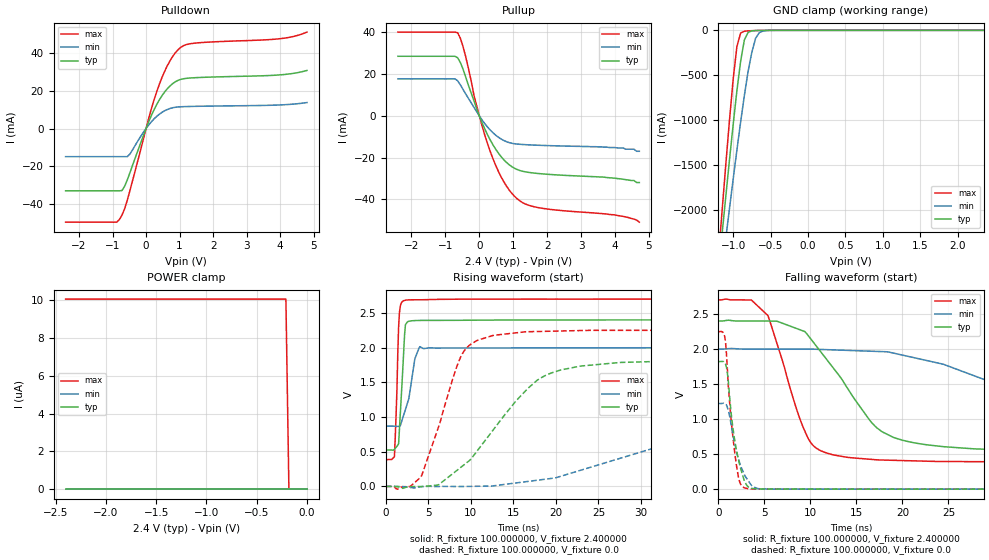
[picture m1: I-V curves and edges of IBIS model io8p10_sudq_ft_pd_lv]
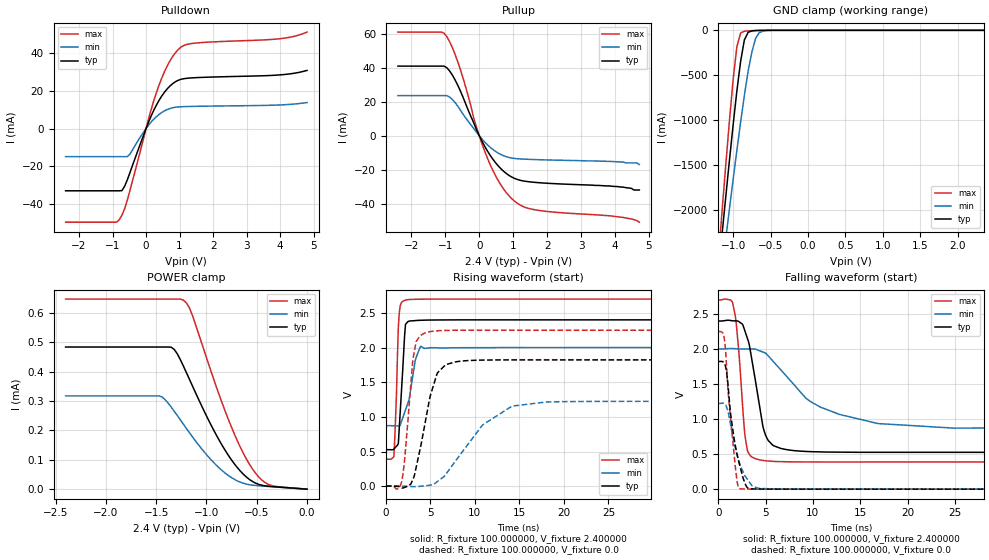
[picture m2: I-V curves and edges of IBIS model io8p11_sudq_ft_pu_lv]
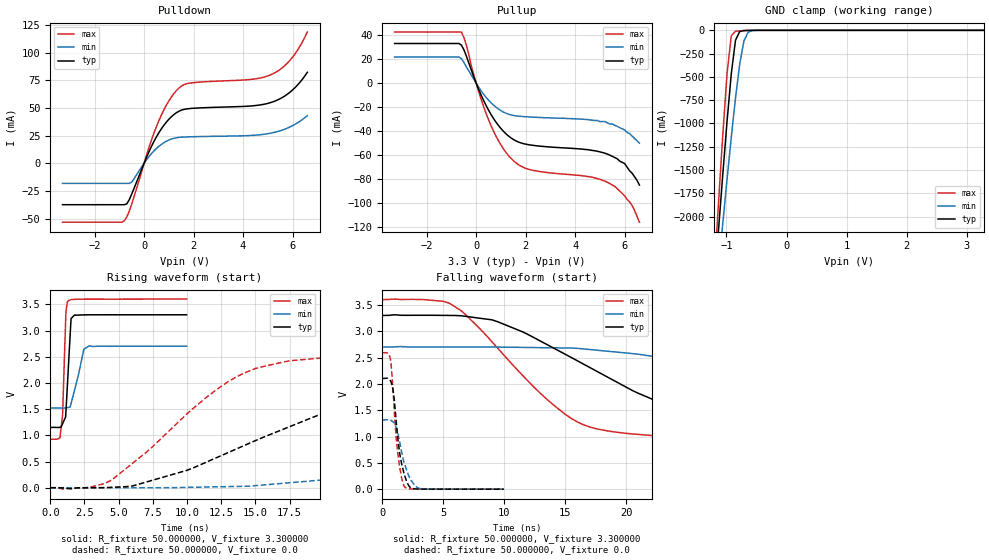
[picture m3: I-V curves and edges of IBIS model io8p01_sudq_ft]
| IBIS file stm32f303x6x8_334_lqfp48.ibs
[IBIS ver] 4.2
[File name] stm32f303x6x8_334_lqfp48.ibs
[File Rev] 1
[Date]  29-09-2025
[Source] Data Created at STMicroelectronics
[Notes]  File originated from ELDO simulations.
[Disclaimer]  This information is for modeling purpose only and is
   not guaranted. The information is subject to change without
   notice.
[Copyright] Copyright 2025 STMicroelectronics Inc.
|   Component stm32f303x6x8_334_lqfp48
[Component] stm32f303x6x8_334_lqfp48
[Manufacturer] STMicroelectronics
[Package]
| variable   typ   min   max
R_pkg   0.0   0.0   0.0
L_pkg   0.0H   0.0H   0.0H
C_pkg   0.0F   0.0F   0.0F
[Pin]  signal_name   model_name   R_pin   L_pin   C_pin
1 VBAT POWER 0.053 3.42534E-09 9.041E-14
2 PC13 io8p_sudq_tc 0.048377332 2.91404E-09 6.443E-14
3 PC14 io8p_sudq_tc 0.044678997 2.50442E-09 4.365E-14
4 PC15 io8p_sudq_tc 0.041905328 2.19704E-09 2.807E-14
5 PF0 io8p_sudq_ft 0.040056325 1.9919E-09 1.769E-14
6 PF1 io8p_sudq_ft 0.03913 1.89021E-09 1.24625E-14
7 NRST ioreset_tc_v33 0.03913 1.89021E-09 1.24625E-14
8 VSSA GND 0.040057312 1.98992E-09 1.775E-14
9 VDDA POWER 0.041906973 2.19374E-09 2.817E-14
10 PA0 io8p_sudq_tc 0.0446813 2.4998E-09 4.379E-14
11 PA1 io8p_sudq_tc 0.048380293 2.9081E-09 6.461E-14
12 PA2 io8p_sudq_tc 0.053 3.42534E-09 9.041E-14
13 PA3 io8p_sudq_tc 0.053 3.42534E-09 9.041E-14
14 PA4 io8p_sudq_tc 0.048377332 2.91404E-09 6.443E-14
15 PA5 io8p_sudq_tc 0.044678997 2.50442E-09 4.365E-14
16 PA6 io8p_sudq_tc 0.041905328 2.19704E-09 2.807E-14
17 PA7 io8p_sudq_tc 0.040056325 1.9919E-09 1.769E-14
18 PB0 io8p_sudq_tc 0.03913 1.89021E-09 1.24625E-14
19 PB1 io8p_sudq_tc 0.03913 1.89021E-09 1.24625E-14
20 PB2 io8p_sudq_tc 0.040057312 1.98992E-09 1.775E-14
21 PB10 io8p_sudq_tc 0.041906973 2.19374E-09 2.817E-14
22 PB11 io8p_sudq_tc 0.0446813 2.4998E-09 4.379E-14
23 VSS GND 0.048380293 2.9081E-09 6.461E-14
24 VDD POWER 0.053 3.42534E-09 9.041E-14
25 PB12 io8p_sudq_tc 0.053 3.42534E-09 9.041E-14
26 PB13 io8p_sudq_tc 0.048377332 2.91404E-09 6.443E-14
27 PB14 io8p_sudq_tc 0.044678997 2.50442E-09 4.365E-14
28 PB15 io8p_sudq_tc 0.041905328 2.19704E-09 2.807E-14
29 PA8 io8p_sudq_ft 0.040056325 1.9919E-09 1.769E-14
30 PA9 io8p_sudq_ft 0.03913 1.89021E-09 1.24625E-14
31 PA10 io8p_sudq_ft 0.03913 1.89021E-09 1.24625E-14
32 PA11 io8p_sudq_ft 0.040057312 1.98992E-09 1.775E-14
33 PA12 io8p_sudq_ft 0.041906973 2.19374E-09 2.817E-14
34 PA13 io8p_sudq_ft 0.0446813 2.4998E-09 4.379E-14
35 VSS GND 0.048380293 2.9081E-09 6.461E-14
36 VDD POWER 0.053 3.42534E-09 9.041E-14
37 PA14 io8p_wsudqh_i2c_ft 0.053 3.42534E-09 9.041E-14
38 PA15 io8p_wsudqh_i2c_ft 0.048377332 2.91404E-09 6.443E-14
39 PB3 io8p_sudq_ft 0.044678997 2.50442E-09 4.365E-14
40 PB4 io8p_sudq_ft 0.041905328 2.19704E-09 2.807E-14
41 PB5 io8p_sudq_ft 0.040056325 1.9919E-09 1.769E-14
42 PB6 io8p_wsudqh_i2c_ft 0.03913 1.89021E-09 1.24625E-14
43 PB7 io8p_wsudqh_i2c_ft 0.03913 1.89021E-09 1.24625E-14
44 BOOT0 vpp_test_hv 0.040057312 1.98992E-09 1.775E-14
45 PB8 io8p_wsudqh_i2c_ft 0.041906973 2.19374E-09 2.817E-14
46 PB9 io8p_wsudqh_i2c_ft 0.0446813 2.4998E-09 4.379E-14
47 VSS_PLUS_1 GND 0.048380293 2.9081E-09 6.461E-14
48 VDD POWER 0.053 3.42534E-09 9.041E-14
[Model Selector] io8p_sudq_ft
io8p01_sudq_ft_pd_lv  "SPEED01 2P0V, PD=40kOhm"
io8p01_sudq_ft_pu_lv  "SPEED01 2P0V, PU=40kOhm"
io8p01_sudq_ft_lv  "SPEED01 2P0V"
io8p10_sudq_ft_pd_lv  "SPEED10 2P0V, PD=40kOhm"
io8p10_sudq_ft_pu_lv  "SPEED10 2P0V, PU=40kOhm"
io8p10_sudq_ft_lv  "SPEED10 2P0V"
io8p11_sudq_ft_pd_lv  "SPEED11 2P0V, PD=40kOhm"
io8p11_sudq_ft_pu_lv  "SPEED11 2P0V, PU=40kOhm"
io8p11_sudq_ft_lv  "SPEED11 2P0V"
io8p01_sudq_ft_pd  "SPEED01, PD=40kOhm"
io8p01_sudq_ft_pu  "SPEED01, PU=40kOhm"
io8p01_sudq_ft  "SPEED01"
io8p10_sudq_ft_pd  "SPEED10, PD=40kOhm"
io8p10_sudq_ft_pu  "SPEED10, PU=40kOhm"
io8p10_sudq_ft  "SPEED10"
io8p11_sudq_ft_pd  "SPEED11, PD=40kOhm"
io8p11_sudq_ft_pu  "SPEED11, PU=40kOhm"
io8p11_sudq_ft  "SPEED11"
[Model Selector] io8p_sudq_tc
io8p01_sudq_tc_pd_lv  "SPEED01 2P0V, PD=40kOhm"
io8p01_sudq_tc_pu_lv  "SPEED01 2P0V, PU=40kOhm"
io8p01_sudq_tc_lv  "SPEED01 2P0V"
io8p10_sudq_tc_pd_lv  "SPEED10 2P0V, PD=40kOhm"
io8p10_sudq_tc_pu_lv  "SPEED10 2P0V, PU=40kOhm"
io8p10_sudq_tc_lv  "SPEED10 2P0V"
io8p11_sudq_tc_pd_lv  "SPEED11 2P0V, PD=40kOhm"
io8p11_sudq_tc_pu_lv  "SPEED11 2P0V, PU=40kOhm"
io8p11_sudq_tc_lv  "SPEED11 2P0V"
io8p01_sudq_tc_pd  "SPEED01, PD=40kOhm"
io8p01_sudq_tc_pu  "SPEED01, PU=40kOhm"
io8p01_sudq_tc  "SPEED01"
io8p10_sudq_tc_pd  "SPEED10, PD=40kOhm"
io8p10_sudq_tc_pu  "SPEED10, PU=40kOhm"
io8p10_sudq_tc  "SPEED10"
io8p11_sudq_tc_pd  "SPEED11, PD=40kOhm"
io8p11_sudq_tc_pu  "SPEED11, PU=40kOhm"
io8p11_sudq_tc  "SPEED11"
[Model Selector] io8p_wsudqh_i2c_ft
io8p_wsudqh_i2c_ft_lv_pd  "General purpose IO with I2C capability on. 5V tolerant. 1.8V range with pull down"
io8p_wsudqh_i2c_ft_lv_pu  "General purpose IO with I2C capability on. 5V tolerant. 1.8V range with pull up"
io8p_wsudqh_i2c_ft_lv  "General purpose IO with I2C capability on. 5V tolerant. 1.8V range"
io8p_wsudqh_i2c_ft_pd  "General purpose IO with I2C capability on. 5V tolerant. 3.3V range with pull down"
io8p_wsudqh_i2c_ft_pu  "General purpose IO with I2C capability on. 5V tolerant. 3.3V range with pull up"
io8p_wsudqh_i2c_ft_i2c  "General purpose IO with I2C capability on. 5V tolerant. 3.3V range"
[Model Selector] ioreset_tc_v33
ioreset_tc_v33_pu_lv  "IORESET 2V + PU=40kOhm"
ioreset_tc_v33_nopu_lv  "IORESET 2V"
ioreset_tc_v33_pu  "IORESET + PU=40kOhm"
ioreset_tc_v33_nopu  "IORESET"
[Model Selector] vpp_test_hv
vpp_test_hv_3p3  "Input Buffer"
vpp_test_hv_2p4  "Input Buffer 2P0V"
| Models and submodels in the file (48): io8p01_sudq_ft_pd_lv (I/O), io8p01_sudq_ft_pu_lv (I/O), io8p01_sudq_ft_lv (I/O), io8p10_sudq_ft_pd_lv (I/O), io8p10_sudq_ft_pu_lv (I/O), io8p10_sudq_ft_lv (I/O), io8p11_sudq_ft_pd_lv (I/O), io8p11_sudq_ft_pu_lv (I/O), io8p11_sudq_ft_lv (I/O), io8p01_sudq_ft_pd (I/O), io8p01_sudq_ft_pu (I/O), io8p01_sudq_ft (I/O), io8p10_sudq_ft_pd (I/O), io8p10_sudq_ft_pu (I/O), io8p10_sudq_ft (I/O), io8p11_sudq_ft_pd (I/O), io8p11_sudq_ft_pu (I/O), io8p11_sudq_ft (I/O), io8p01_sudq_tc_pd_lv (I/O), io8p01_sudq_tc_pu_lv (I/O), io8p01_sudq_tc_lv (I/O), io8p10_sudq_tc_pd_lv (I/O), io8p10_sudq_tc_pu_lv (I/O), io8p10_sudq_tc_lv (I/O), io8p11_sudq_tc_pd_lv (I/O), io8p11_sudq_tc_pu_lv (I/O), io8p11_sudq_tc_lv (I/O), io8p01_sudq_tc_pd (I/O), io8p01_sudq_tc_pu (I/O), io8p01_sudq_tc (I/O), io8p10_sudq_tc_pd (I/O), io8p10_sudq_tc_pu (I/O), io8p10_sudq_tc (I/O), io8p11_sudq_tc_pd (I/O), io8p11_sudq_tc_pu (I/O), io8p11_sudq_tc (I/O), io8p_wsudqh_i2c_ft_lv_pd (I/O), io8p_wsudqh_i2c_ft_lv_pu (I/O), io8p_wsudqh_i2c_ft_lv (I/O), io8p_wsudqh_i2c_ft_pd (I/O), io8p_wsudqh_i2c_ft_pu (I/O), io8p_wsudqh_i2c_ft_i2c (I/O), ioreset_tc_v33_pu_lv (I/O_open_drain), ioreset_tc_v33_nopu_lv (I/O_open_drain), ioreset_tc_v33_pu (I/O_open_drain), ioreset_tc_v33_nopu (I/O_open_drain), vpp_test_hv_2p4 (Input), vpp_test_hv_3p3 (Input)
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|   Model io8p10_sudq_ft_pd_lv
[Model]  io8p10_sudq_ft_pd_lv
Model_type I/O
Polarity   Non-Inverting
Enable   Active-Low
Vinl =   0.720000V
Vinh =   1.680000V
Vmeas =  1.200000V
Cref =   50.000000pF
Rref =   100.000000M
Vref =   0.0V
C_comp   1.970100pF   1.887900pF   2.069400pF
[Temperature Range]   25.000000   0.125000k   -40.000000
[Pullup Reference]   2.400000V   2.000000V   2.700000V
[Pulldown Reference]   0.0V   0.0V   0.0V
[POWER Clamp Reference]   2.400000V   2.000000V   2.700000V
[GND Clamp Reference]   0.0V   0.0V   0.0V
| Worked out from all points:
|   slope of the pulldown table from 0 to 0.36 V, typ, clamps not added: 25.5 ohm
|   slope of the pullup table from 0 to 0.36 V, typ, clamps not added: 28.4 ohm
|   GND clamp passes 1 mA (typ) near -0.64 V on its own axis
|   rising waveform, R_fixture 100.000000, V_fixture 2.400000: 20-80 % time 501ps typ, 1.06ns min, 337ps max; typ from 0.525 V to 2.4 V
|   rising waveform, R_fixture 100.000000, V_fixture 0.0: 20-80 % time 7.37ns typ, 21.8ns min, 3.53ns max; typ from 0 V to 1.82 V
|   falling waveform, R_fixture 100.000000, V_fixture 2.400000: 20-80 % time 6.27ns typ, 17.5ns min, 3.34ns max; typ from 2.4 V to 0.525 V
|   falling waveform, R_fixture 100.000000, V_fixture 0.0: 20-80 % time 1.15ns typ, 1.39ns min, 910ps max; typ from 1.82 V to 0 V
[Pulldown]
|Voltage   I(typ)   I(min)   I(max)
-2.4V     -33.16mA   -14.98mA   -49.86mA
-880mV    -33.16mA   -14.98mA   -49.86mA
-800mV    -33.16mA   -14.98mA   -48.55mA
-640mV    -30.75mA   -14.98mA   -42.76mA
-480mV    -23.43mA   -13.57mA   -32.92mA
80mV      3.651mA    1.905mA    5.506mA
400mV     15.37mA    7.665mA    23.73mA
720mV     22.75mA    10.69mA    36.23mA
1.04V     26.18mA    11.57mA    43.27mA
1.52V     27.09mA    11.81mA    45.55mA
4V        28.55mA    12.55mA    47.81mA
4.8V      30.9mA     13.81mA    51.31mA
[Pullup]
|Voltage   I(typ)   I(min)   I(max)
-2.4V     28.56mA    17.75mA    40.16mA
-720mV    28.56mA    17.75mA    40.16mA
-640mV    27.85mA    16.83mA    39.87mA
-480mV    22.39mA    12.66mA    33.22mA
-80mV     3.427mA    2.067mA    4.957mA
160mV     -6.219mA   -3.715mA   -9.137mA
320mV     -11.51mA   -6.781mA   -16.98mA
720mV     -21mA      -11.8mA    -31.53mA
1.12V     -25.77mA   -13.54mA   -39.82mA
1.76V     -27.69mA   -14.12mA   -44.07mA
4V        -29.9mA    -15.2mA    -47.5mA
4.72V     -32mA      -17mA      -51mA
[GND_clamp]
|Voltage   I(typ)   I(min)   I(max)
-2.4V     -9.788A    -9.782A    -9.734A
-1.2V     -2.718A    -3.021A    -2.568A
-1.15V    -2.29A     -2.675A    -2.036A
-1.1V     -1.868A    -2.333A    -1.515A
-1.05V    -1.454A    -1.995A    -1.012A
-950mV    -674.5mA   -1.337A    -180.6mA
-900mV    -345.2mA   -1.023A    -29.74mA
-850mV    -106.4mA   -726mA     -10.14mA
-750mV    -6.411mA   -244mA     -4.042mA
-700mV    -2.572mA   -88.62mA   -2.346mA
-600mV    -429.6uA   -7.75mA    -383.5uA
2.35V     59.77uA    46.33uA    66.89uA
[POWER_clamp]
|Voltage   I(typ)   I(min)   I(max)
-2.4V     0A         0A         10.06uA
-210mV    0A         0A         10.06uA
-180mV    0A         0A         0A
0V        0A         0A         0A
[Ramp]
| variable   typ   min   max
dV/dt_r  1.09206/7.36205n   0.73212/21.76780n   1.34880/3.52140n
dV/dt_f  1.12434/6.26286n   0.67629/17.46251n   1.38699/3.33301n
R_load = 100.000000
[Rising Waveform]
R_fixture= 100.000000
V_fixture= 2.400000
V_fixture_min= 2.000000
V_fixture_max= 2.700000
|time   V(typ)   V(min)   V(max)
0s        524.8mV    868.7mV    387.2mV
1.001ns   532.8mV    867mV      426.6mV
1.301ns   578.6mV    865.5mV    1.387V
1.502ns   616.5mV    864.9mV    2.303V
1.702ns   1.053V     875.4mV    2.602V
2.102ns   1.953V     1.031V     2.676V
2.302ns   2.331V     1.108V     2.683V
3.403ns   2.389V     1.835V     2.689V
4.004ns   2.392V     2.014V     2.689V
49.85ns   2.399V     1.999V     2.699V
[Rising Waveform]
R_fixture= 100.000000
V_fixture= 0.0
V_fixture_min= 0.0
V_fixture_max= 0.0
|time   V(typ)   V(min)   V(max)
0s        1.768nV    15.89nV    1.355nV
2.803ns   -3.26mV    -14.06mV   -1.551mV
4.204ns   -1.822mV   -2.484mV   153.2mV
6.206ns   24.43mV    -1.172mV   860.8mV
8.809ns   274.4mV    -1.373mV   1.867V
12.61ns   812.3mV    7.914mV    2.175V
17.82ns   1.532V     89.58mV    2.232V
23.02ns   1.735V     237.2mV    2.246V
50.05ns   1.82V      1.08V      2.248V
99.7ns    1.82V      1.221V     2.248V
[Falling Waveform]
R_fixture= 100.000000
V_fixture= 2.400000
V_fixture_min= 2.000000
V_fixture_max= 2.700000
|time   V(typ)   V(min)   V(max)
0s        2.399V     1.999V     2.699V
3.604ns   2.399V     1.998V     2.698V
5.405ns   2.398V     1.998V     2.475V
9.61ns    2.218V     1.997V     767.5mV
12.61ns   1.708V     1.986V     485.9mV
17.62ns   835.2mV    1.963V     416.1mV
24.42ns   606.3mV    1.782V     394.4mV
31.83ns   557.1mV    1.421V     389.7mV
47.25ns   529mV      987.2mV    387.3mV
99.7ns    524.8mV    868.7mV    387.2mV
[Falling Waveform]
R_fixture= 100.000000
V_fixture= 0.0
V_fixture_min= 0.0
V_fixture_max= 0.0
|time   V(typ)   V(min)   V(max)
0s        1.82V      1.221V     2.248V
700.7ps   1.8V       1.221V     2.179V
800.8ps   1.783V     1.214V     2.096V
1.001ns   1.653V     1.163V     1.703V
1.401ns   1.09V      921.9mV    991.5mV
1.802ns   688.2mV    647.3mV    514.6mV
2.302ns   364.8mV    386.2mV    116.7mV
2.903ns   104.8mV    188.7mV    16.24mV
4.705ns   2.13mV     3.846mV    2.055mV
49.85ns   1.768nV    15.89nV    1.355nV
|   Model io8p11_sudq_ft_pu_lv
[Model]  io8p11_sudq_ft_pu_lv
Model_type I/O
Polarity   Non-Inverting
Enable   Active-Low
Vinl =   0.720000V
Vinh =   1.680000V
Vmeas =  1.200000V
Cref =   50.000000pF
Rref =   100.000000M
Vref =   0.0V
C_comp   1.970100pF   1.887900pF   2.069400pF
[Temperature Range]   25.000000   0.125000k   -40.000000
[Pullup Reference]   2.400000V   2.000000V   2.700000V
[Pulldown Reference]   0.0V   0.0V   0.0V
[POWER Clamp Reference]   2.400000V   2.000000V   2.700000V
[GND Clamp Reference]   0.0V   0.0V   0.0V
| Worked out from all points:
|   slope of the pulldown table from 0 to 0.36 V, typ, clamps not added: 25.5 ohm
|   slope of the pullup table from 0 to 0.36 V, typ, clamps not added: 28.4 ohm
|   GND clamp passes 1 mA (typ) near -0.64 V on its own axis
|   rising waveform, R_fixture 100.000000, V_fixture 2.400000: 20-80 % time 508ps typ, 1.05ns min, 337ps max; typ from 0.527 V to 2.4 V
|   rising waveform, R_fixture 100.000000, V_fixture 0.0: 20-80 % time 1.8ns typ, 4.87ns min, 863ps max; typ from 0.001 V to 1.82 V
|   falling waveform, R_fixture 100.000000, V_fixture 2.400000: 20-80 % time 1.39ns typ, 6.08ns min, 775ps max; typ from 2.4 V to 0.527 V
|   falling waveform, R_fixture 100.000000, V_fixture 0.0: 20-80 % time 1.17ns typ, 1.4ns min, 853ps max; typ from 1.82 V to 0.001 V
[Pulldown]
|Voltage   I(typ)   I(min)   I(max)
-2.4V     -33.16mA   -14.98mA   -49.86mA
-880mV    -33.16mA   -14.98mA   -49.86mA
-800mV    -33.16mA   -14.98mA   -48.55mA
-640mV    -30.75mA   -14.98mA   -42.77mA
-480mV    -23.43mA   -13.57mA   -32.92mA
80mV      3.651mA    1.905mA    5.506mA
400mV     15.37mA    7.665mA    23.73mA
720mV     22.75mA    10.69mA    36.23mA
1.04V     26.18mA    11.57mA    43.27mA
1.52V     27.09mA    11.81mA    45.55mA
4V        28.55mA    12.55mA    47.81mA
4.8V      30.9mA     13.81mA    51.31mA
[Pullup]
|Voltage   I(typ)   I(min)   I(max)
-2.4V     41.12mA    23.71mA    61.21mA
-1.12V    41.12mA    23.71mA    61.21mA
-960mV    40.18mA    23.71mA    58.56mA
-800mV    36.01mA    21.55mA    52.29mA
-560mV    26.54mA    15.18mA    39.21mA
-160mV    7.421mA    4.162mA    10.02mA
240mV     -8.977mA   -5.327mA   -13.21mA
640mV     -19.51mA   -11.09mA   -29.16mA
1.04V     -25.15mA   -13.38mA   -38.61mA
1.68V     -27.56mA   -14.07mA   -43.82mA
3.84V     -29.6mA    -15.1mA    -47.2mA
4.72V     -32mA      -17mA      -51mA
[GND_clamp]
|Voltage   I(typ)   I(min)   I(max)
-2.4V     -9.788A    -9.782A    -9.734A
-1.2V     -2.718A    -3.02A     -2.568A
-1.15V    -2.29A     -2.675A    -2.036A
-1.1V     -1.868A    -2.333A    -1.515A
-1.05V    -1.454A    -1.995A    -1.012A
-950mV    -674.5mA   -1.337A    -180.5mA
-900mV    -345.2mA   -1.023A    -29.72mA
-850mV    -106.4mA   -726mA     -10.13mA
-750mV    -6.396mA   -244mA     -4.026mA
-700mV    -2.558mA   -88.61mA   -2.329mA
-600mV    -416uA     -7.739mA   -368uA
2.35V     0A         0A         0A
[POWER_clamp]
|Voltage   I(typ)   I(min)   I(max)
-2.4V     483.8uA    317.4uA    647uA
-1.47V    483.8uA    317.4uA    647uA
-1.32V    475.6uA    265.2uA    647uA
-1.23V    419.7uA    221.6uA    643.3uA
-1.17V    374.8uA    192.7uA    617.6uA
-1.14V    352.1uA    178.7uA    591.9uA
-840mV    147uA      62.15uA    289.6uA
-690mV    72.24uA    27.76uA    162.7uA
-540mV    25.74uA    13.55uA    67.63uA
-450mV    13.38uA    10.75uA    31.36uA
-360mV    9.231uA    8.535uA    12.97uA
0V        0A         0A         0A
[Ramp]
| variable   typ   min   max
dV/dt_r  1.09269/1.79328n   0.73359/4.86832n   1.34926/0.85997n
dV/dt_f  1.12411/1.38607n   0.67669/6.07307n   1.38681/0.77427n
R_load = 100.000000
[Rising Waveform]
R_fixture= 100.000000
V_fixture= 2.400000
V_fixture_min= 2.000000
V_fixture_max= 2.700000
|time   V(typ)   V(min)   V(max)
0s        526.5mV    872.5mV    388.6mV
900.9ps   534.2mV    870.9mV    425.1mV
1.201ns   577.4mV    869.6mV    1.365V
1.401ns   613.7mV    869.2mV    2.295V
1.602ns   1.046V     879.2mV    2.598V
2.202ns   2.333V     1.099V     2.686V
2.603ns   2.381V     1.245V     2.693V
3.303ns   2.389V     1.817V     2.697V
3.904ns   2.394V     2.019V     2.698V
49.85ns   2.4V       2V         2.7V
[Rising Waveform]
R_fixture= 100.000000
V_fixture= 0.0
V_fixture_min= 0.0
V_fixture_max= 0.0
|time   V(typ)   V(min)   V(max)
0s        1.022mV    1.341mV    911uV
1.802ns   -26.21mV   109.9uV    74.5mV
3.103ns   116.7mV    -6.8mV     1.877V
3.403ns   271.6mV    -8.185mV   2.086V
4.505ns   979.1mV    4.99mV     2.215V
5.706ns   1.605V     58.19mV    2.241V
6.707ns   1.752V     167.1mV    2.247V
10.81ns   1.819V     875.7mV    2.25V
14.21ns   1.822V     1.156V     2.25V
49.85ns   1.822V     1.224V     2.25V
[Falling Waveform]
R_fixture= 100.000000
V_fixture= 2.400000
V_fixture_min= 2.000000
V_fixture_max= 2.700000
|time   V(typ)   V(min)   V(max)
0s        2.4V       2V         2.7V
1.502ns   2.403V     2.008V     2.671V
1.902ns   2.401V     2.004V     2.37V
2.903ns   2.224V     2.001V     697.7mV
4.004ns   1.486V     1.995V     432.1mV
5.205ns   712.7mV    1.914V     402.8mV
7.508ns   558.9mV    1.567V     391mV
10.81ns   532.3mV    1.17V      388.6mV
16.82ns   526.7mV    938mV      388.6mV
49.85ns   526.5mV    872.5mV    388.6mV
[Falling Waveform]
R_fixture= 100.000000
V_fixture= 0.0
V_fixture_min= 0.0
V_fixture_max= 0.0
|time   V(typ)   V(min)   V(max)
0s        1.822V     1.224V     2.25V
700.7ps   1.784V     1.216V     2.102V
1.101ns   1.384V     1.072V     1.307V
1.301ns   1.083V     926.1mV    1.012V
1.802ns   627.4mV    595.9mV    327.6mV
2.102ns   434.5mV    435.4mV    35.99mV
2.302ns   325.6mV    349.7mV    5.728mV
3.103ns   17.78mV    137.1mV    2.333mV
4.605ns   2.394mV    9.48mV     1.404mV
49.85ns   1.022mV    1.341mV    911uV
|   Model io8p01_sudq_ft
[Model]  io8p01_sudq_ft
Model_type I/O
Polarity   Non-Inverting
Enable   Active-Low
Vinl =   0.990000V
Vinh =   2.310000V
Vmeas =  1.650000V
Cref =   50.000000pF
Rref =   100.000000M
Vref =   0.0V
C_comp   1.970900pF   1.892300pF   2.063200pF
[Temperature Range]   25.000000   0.125000k   -40.000000
[Pullup Reference]   3.300000V   2.700000V   3.600000V
[Pulldown Reference]   0.0V   0.0V   0.0V
[POWER Clamp Reference]   3.300000V   2.700000V   3.600000V
[GND Clamp Reference]   0.0V   0.0V   0.0V
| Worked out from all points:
|   slope of the pulldown table from 0 to 0.495 V, typ, clamps not added: 20.9 ohm
|   slope of the pullup table from 0 to 0.495 V, typ, clamps not added: 22.2 ohm
|   GND clamp passes 1 mA (typ) near -0.64 V on its own axis
|   rising waveform, R_fixture 50.000000, V_fixture 3.300000: 20-80 % time 269ps typ, 640ps min, 200ps max; typ from 1.15 V to 3.3 V
|   rising waveform, R_fixture 50.000000, V_fixture 0.0: 20-80 % time 12.5ns typ, 30.4ns min, 7.06ns max; typ from 0 V to 2.1 V
|   falling waveform, R_fixture 50.000000, V_fixture 3.300000: 20-80 % time 10.9ns typ, 22.8ns min, 6.88ns max; typ from 3.3 V to 1.15 V
|   falling waveform, R_fixture 50.000000, V_fixture 0.0: 20-80 % time 666ps typ, 862ps min, 543ps max; typ from 2.1 V to 0 V
[Pulldown]
|Voltage   I(typ)   I(min)   I(max)
-3.3V     -37.45mA   -18.2mA    -53.24mA
-800mV    -37.45mA   -18.2mA    -51.9mA
-700mV    -36.7mA    -18.2mA    -48.48mA
-500mV    -27.71mA   -17.01mA   -36.66mA
200mV     10.57mA    6.084mA    14.57mA
500mV     23.91mA    13.38mA    33.24mA
900mV     37.17mA    19.88mA    52.48mA
1.3V      45.55mA    23.01mA    65.5mA
1.8V      49.29mA    23.83mA    72.18mA
5.1V      54.68mA    27.07mA    79.72mA
5.9V      64.2mA     32.82mA    93.01mA
6.6V      82.13mA    42.97mA    118.4mA
[Pullup]
|Voltage   I(typ)   I(min)   I(max)
-3.3V     33.18mA    21.9mA     42.7mA
-600mV    31.87mA    20.57mA    42.7mA
-400mV    22.78mA    13.76mA    31.89mA
100mV     -5.13mA    -3.299mA   -6.952mA
500mV     -22.5mA    -14.16mA   -30.52mA
900mV     -35.28mA   -21.55mA   -48mA
1.4V      -45.55mA   -26.41mA   -62.54mA
2.2V      -51.57mA   -28.22mA   -72.25mA
5.4V      -60mA      -34mA      -83.7mA
6V        -67mA      -39mA      -94mA
6.2V      -73mA      -42mA      -99mA
6.6V      -85mA      -50mA      -116mA
[GND_clamp]
|Voltage   I(typ)   I(min)   I(max)
-3.3V     -9.525A    -9.501A    -9.513A
-1.2V     -2.719A    -3.023A    -2.568A
-1.13V    -2.122A    -2.541A    -1.826A
-1.06V    -1.537A    -2.065A    -1.111A
-990mV    -975.7mA   -1.599A    -462mA
-920mV    -467.4mA   -1.149A    -59mA
-850mV    -106.6mA   -727.3mA   -10.11mA
-780mV    -13.06mA   -365.4mA   -5.254mA
-710mV    -3.045mA   -114.8mA   -2.635mA
-640mV    -943.2uA   -20.16mA   -905.7uA
-570mV    -199.4uA   -3.959mA   -156.8uA
3.28V     0A         0A         0A
[POWER_clamp]
|Voltage   I(typ)   I(min)   I(max)
-3.28V    0A         0A         0A
0V        0A         0A         0A
[Ramp]
| variable   typ   min   max
dV/dt_r  1.26240/12.53718n   0.78948/30.37625n   1.55460/7.05051n
dV/dt_f  1.28952/10.93890n   0.70650/22.81705n   1.60469/6.86180n
R_load = 50.000000
[Rising Waveform]
R_fixture= 50.000000
V_fixture= 3.300000
V_fixture_min= 2.700000
V_fixture_max= 3.600000
|time   V(typ)   V(min)   V(max)
0s        1.151V     1.522V     925.5mV
720.7ps   1.153V     1.522V     979.3mV
900.9ps   1.222V     1.52V      1.393V
1.141ns   1.422V     1.523V     3.312V
1.261ns   1.999V     1.529V     3.554V
1.522ns   3.228V     1.605V     3.588V
1.762ns   3.294V     1.851V     3.595V
2.462ns   3.298V     2.646V     3.599V
2.863ns   3.3V       2.708V     3.599V
9.97ns    3.3V       2.7V       3.6V
[Rising Waveform]
R_fixture= 50.000000
V_fixture= 0.0
V_fixture_min= 0.0
V_fixture_max= 0.0
|time   V(typ)   V(min)   V(max)
0s        2.028nV    11.57nV    2.55nV
4.505ns   8.246mV    23.61uV    149.8mV
10.01ns   333.3mV    6.624mV    1.413V
14.01ns   785.5mV    26.06mV    2.168V
22.52ns   1.625V     206.1mV    2.53V
28.03ns   1.898V     345.1mV    2.568V
39.54ns   2.061V     685.1mV    2.588V
55.56ns   2.101V     1.054V     2.592V
75.08ns   2.103V     1.24V      2.591V
249.2ns   2.104V     1.316V     2.591V
[Falling Waveform]
R_fixture= 50.000000
V_fixture= 3.300000
V_fixture_min= 2.700000
V_fixture_max= 3.600000
|time   V(typ)   V(min)   V(max)
0s        3.3V       2.7V       3.6V
5.506ns   3.3V       2.701V     3.532V
9.009ns   3.216V     2.7V       2.797V
13.01ns   2.808V     2.688V     1.811V
16.02ns   2.437V     2.675V     1.275V
22.52ns   1.673V     2.511V     1.015V
30.53ns   1.307V     2.227V     958.1mV
45.05ns   1.189V     1.779V     932.1mV
69.57ns   1.157V     1.587V     925.7mV
249.2ns   1.151V     1.522V     925.5mV
[Falling Waveform]
R_fixture= 50.000000
V_fixture= 0.0
V_fixture_min= 0.0
V_fixture_max= 0.0
|time   V(typ)   V(min)   V(max)
0s        2.104V     1.316V     2.591V
660.7ps   2.062V     1.315V     2.466V
900.9ps   1.84V      1.273V     1.796V
1.141ns   1.275V     1.165V     952.9mV
1.261ns   977.3mV    1.075V     694.5mV
1.602ns   464.8mV    685.7mV    192.5mV
1.862ns   238.4mV    452mV      36.35mV
2.282ns   34.71mV    203.8mV    5.722mV
3.103ns   2.027mV    11.23mV    1.089mV
9.97ns    2.028nV    11.57nV    2.55nV
